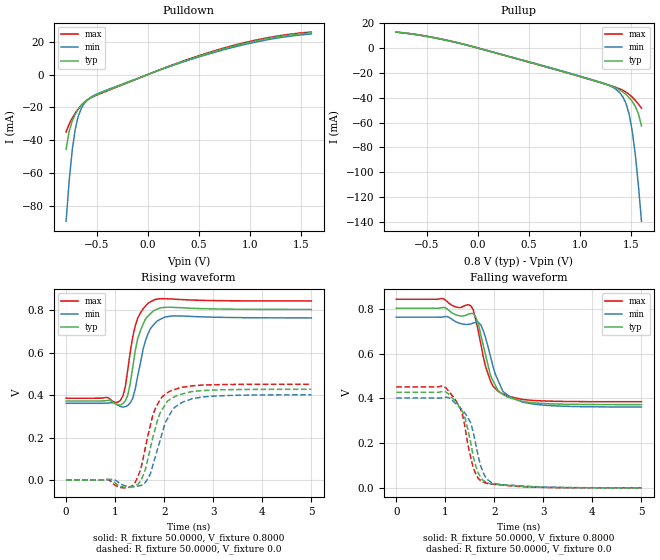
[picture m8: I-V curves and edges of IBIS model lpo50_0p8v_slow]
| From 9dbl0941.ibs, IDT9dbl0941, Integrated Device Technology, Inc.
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|   Model lpo50_0p8v_slow
[Model]  lpo50_0p8v_slow
Model_type Output
Polarity   Non-Inverting
Vmeas =  0.4000V
Cref =   2.0000pF
Rref =   0.0
Vref =   0.4000V
C_comp   1.1000pF   1.0000pF   1.2000pF
[Temperature Range]   27.0000   70.0000   0.0
[Voltage Range]   0.8000V   0.7600V   0.8400V
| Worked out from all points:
|   slope of the pulldown table from 0 to 0.12 V, typ, clamps not added: 41.4 ohm
|   slope of the pullup table from 0 to 0.12 V, typ, clamps not added: 44.4 ohm
|   rising waveform, R_fixture 50.0000, V_fixture 0.8000: 20-80 % time 229ps typ, 240ps min, 215ps max; typ from 0.372 V to 0.804 V
|   rising waveform, R_fixture 50.0000, V_fixture 0.0: 20-80 % time 332ps typ, 362ps min, 315ps max; typ from 0 V to 0.428 V
|   falling waveform, R_fixture 50.0000, V_fixture 0.8000: 20-80 % time 332ps typ, 349ps min, 302ps max; typ from 0.804 V to 0.373 V
|   falling waveform, R_fixture 50.0000, V_fixture 0.0: 20-80 % time 295ps typ, 312ps min, 279ps max; typ from 0.428 V to 0 V
[Pulldown]
|Voltage   I(typ)   I(min)   I(max)
-800mV    -45.52mA   -89.42mA   -34.99mA
-770mV    -34.69mA   -64.98mA   -30.13mA
-740mV    -28.29mA   -46.11mA   -26.53mA
-710mV    -24.18mA   -33.19mA   -23.49mA
-680mV    -21.17mA   -25.25mA   -20.86mA
-650mV    -18.77mA   -20.52mA   -18.63mA
-620mV    -16.84mA   -17.54mA   -16.82mA
-560mV    -14.08mA   -14mA      -14.27mA
100mV     2.426mA    2.317mA    2.503mA
670mV     14.39mA    13.82mA    14.78mA
1.15V     21.69mA    20.96mA    22.14mA
1.6V      25.43mA    24.71mA    25.88mA
[Pullup]
|Voltage   I(typ)   I(min)   I(max)
-800mV    12.69mA    12.68mA    12.51mA
-440mV    8.345mA    8.179mA    8.402mA
-20mV     274.7uA    267.5uA    282.2uA
1.15V     -26.68mA   -26.4mA    -26.75mA
1.36V     -32.54mA   -33.95mA   -32.08mA
1.42V     -35.56mA   -39.7mA    -34.16mA
1.45V     -37.62mA   -44.96mA   -35.6mA
1.48V     -40.1mA    -53.57mA   -37.41mA
1.51V     -43.12mA   -67.09mA   -39.62mA
1.54V     -47.08mA   -86.23mA   -42.2mA
1.57V     -53mA      -110.6mA   -45.14mA
1.6V      -62.75mA   -139.3mA   -48.48mA
[Ramp]
| variable   typ   min   max
dV/dt_r  0.2567/0.3320n   0.2411/0.3621n   0.2710/0.3149n
dV/dt_f  0.2589/0.3315n   0.2413/0.3492n   0.2750/0.3019n
R_load = 50.0000
[Rising Waveform]
R_fixture= 50.0000
V_fixture= 0.8000
V_fixture_min= 0.7600
V_fixture_max= 0.8400
|time   V(typ)   V(min)   V(max)
0s        372.5mV    361.7mV    385.7mV
1.11ns    354.2mV    346.3mV    376.6mV
1.21ns    373.9mV    346.2mV    443.6mV
1.26ns    401.2mV    352.1mV    522.8mV
1.36ns    533.9mV    386.2mV    676.1mV
1.46ns    666.4mV    490.2mV    762.7mV
1.62ns    759.3mV    657.9mV    820.2mV
1.82ns    802.3mV    740.8mV    851.5mV
2.17ns    814.1mV    773.6mV    853.1mV
5ns       804.2mV    764.1mV    844.1mV
[Rising Waveform]
R_fixture= 50.0000
V_fixture= 0.0
V_fixture_min= 0.0
V_fixture_max= 0.0
|time   V(typ)   V(min)   V(max)
0s        0V         0V         0V
960ps     -5.271mV   3.093mV    -17.63mV
1.36ns    -31.53mV   -32.18mV   -24.98mV
1.52ns    -5.139mV   -25.79mV   49.05mV
1.72ns    152.5mV    30.63mV    259.5mV
1.92ns    318.3mV    189.8mV    380.5mV
2.12ns    379.9mV    311.1mV    419.4mV
2.37ns    405.7mV    366.6mV    437.5mV
2.78ns    421.3mV    391mV      447.6mV
5ns       427.8mV    401.9mV    451.6mV
[Falling Waveform]
R_fixture= 50.0000
V_fixture= 0.8000
V_fixture_min= 0.7600
V_fixture_max= 0.8400
|time   V(typ)   V(min)   V(max)
0s        804.1mV    764mV      844.1mV
1.01ns    804.9mV    767.1mV    839.4mV
1.52ns    780.5mV    733.3mV    815.2mV
1.62ns    764.9mV    740.5mV    752.7mV
1.72ns    688.5mV    731.2mV    647.6mV
1.92ns    503.7mV    588.4mV    478.4mV
2.17ns    419.3mV    433.5mV    421.1mV
2.27ns    406.2mV    415.6mV    411.3mV
3.03ns    377.4mV    369.7mV    388.8mV
5ns       372.6mV    361.8mV    385.7mV
[Falling Waveform]
R_fixture= 50.0000
V_fixture= 0.0
V_fixture_min= 0.0
V_fixture_max= 0.0
|time   V(typ)   V(min)   V(max)
0s        427.8mV    402mV      451.7mV
1.01ns    429.7mV    405.7mV    448mV
1.31ns    356mV      357.1mV    352.4mV
1.41ns    307.2mV    331.7mV    260.1mV
1.52ns    201mV      289.7mV    134.1mV
1.62ns    98.25mV    196.2mV    62.96mV
1.77ns    32.88mV    69.47mV    25.16mV
1.92ns    18.81mV    27.05mV    16.93mV
2.17ns    13.03mV    14.13mV    11.8mV
5ns       18.13uV    53.61uV    7.647uV
